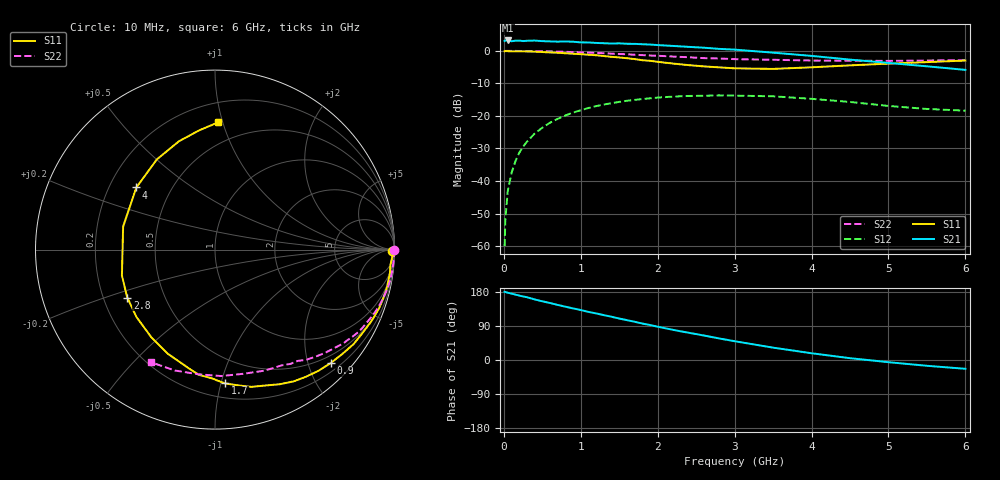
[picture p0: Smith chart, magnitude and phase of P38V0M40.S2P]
! SIEMENS Small Signal Semiconductors
! BFP181
! Si NPN RF Bipolar Junction Transistor in SOT143
! VCE = 8 V  IC = 0.4 mA
! Common Emitter S-Parameters:  March  1996
# GHz  S  MA  R  50
!  f  S11  S21  S12  S22
! GHz  MAG  ANG  MAG  ANG  MAG  ANG  MAG  ANG
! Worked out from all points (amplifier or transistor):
!   36 points, 10 MHz to 6 GHz, reference 50 ohm
!   highest |S21| = 3.2 dB at 50 MHz (marker M1)
!   |S21| within 3 dB of that: start of sweep to 3.1 GHz
!   unconditionally stable (mu >= 1): 3.935 GHz to end of sweep
!   at 250 MHz: K = 0.08, MSG = 16.2 dB, |S12| = -29.5 dB
!   at 1.4 GHz: K = 0.42, MSG = 9.2 dB, |S12| = -16.1 dB
!   at 6 GHz: K = 1.47, MAG = 2.2 dB, |S12| = -18.4 dB
!   S11 on the Smith chart (normalised r, x): 10 MHz: open; 900 MHz: 0.35, -2.40; 1.7 GHz: 0.30, -1.03; 2.8 GHz: 0.30, -0.23; 4 GHz: 0.31, +0.32; 6 GHz: 0.34, +0.97
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0.01  0.9857 -0.6  1.418 179.8  0.001 76.8  1 -0.2
0.02  0.994 -1.2  1.442 179.6  0.0026 86.4  0.996 -0.4
0.05  0.9887 -2.2  1.443 177.5  0.0069 91.7  0.9978 -1.2
0.1  0.9811 -5.0  1.404 175.2  0.0133 85.4  0.9982 -2.5
0.15  0.9834 -7.6  1.43 172.6  0.0201 84.5  0.9968 -3.7
0.2  0.9813 -9.9  1.435 170.0  0.0271 82.8  0.9955 -5.0
0.3  0.9773 -14.8  1.426 165.7  0.0402 79.2  0.9935 -7.4
0.4  0.9713 -19.6  1.438 159.9  0.0535 75.9  0.9909 -9.8
0.6  0.9441 -29.5  1.396 150.4  0.0786 68.0  0.9793 -14.6
0.9  0.9027 -44.5  1.38 136.1  0.1127 57.5  0.956 -21.6
1.1  0.871 -54.4  1.345 126.9  0.1325 50.9  0.937 -26.0
1.5  0.791 -75.2  1.303 109.4  0.1643 38.4  0.8942 -34.3
1.7  0.7474 -85.8  1.279 100.9  0.1763 32.5  0.8709 -38.2
1.9  0.7034 -97.4  1.249 92.3  0.1866 26.8  0.8483 -41.8
2.2  0.6372 -114.3  1.188 79.5  0.1981 19.1  0.8172 -47.0
2.8  0.5572 -151.3  1.071 56.8  0.207 4.9  0.7629 -56.6
3  0.5384 -164.4  1.044 49.6  0.2052 0.3  0.745 -59.9
3.5  0.5278 165.9  0.937 32.6  0.2003 -9.3  0.7286 -67.8
4  0.5584 141.7  0.836 17.8  0.1832 -17.2  0.7097 -77.1
4.5  0.598 122.8  0.733 4.8  0.164 -23.1  0.7054 -87.2
5.5  0.6704 97.5  0.578 -15.3  0.128 -22.3  0.7096 -108.3
6  0.7093 88.6  0.51 -23.2  0.1205 -18.1  0.7214 -119.4
